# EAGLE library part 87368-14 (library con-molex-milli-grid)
RECEPTACAL
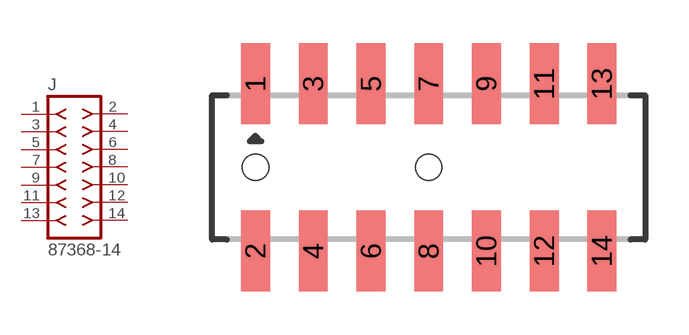
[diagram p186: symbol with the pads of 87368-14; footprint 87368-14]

Designator prefix J

## 87368-14  [87368-14]
1  1  pas
2  2  pas
3  3  pas
4  4  pas
5  5  pas
6  6  pas
7  7  pas
8  8  pas
9  9  pas
10  10  pas
11  11  pas
12  12  pas
13  13  pas
14  14  pas

## Footprint 87368-14 (pad centres in mm)
RECEPTACAL SMD Dual Row, Side Entry
smd 1 x 2.8: 1 -6,2.9; 2 -6,-2.9; 3 -4,2.9; 4 -4,-2.9; 5 -2,2.9; 6 -2,-2.9; 7 0,2.9; 8 0,-2.9; 9 2,2.9; 10 2,-2.9; 11 4,2.9; 12 4,-2.9; 13 6,2.9; 14 6,-2.9
hole 0.914 at -6,0
hole 0.914 at 0,0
